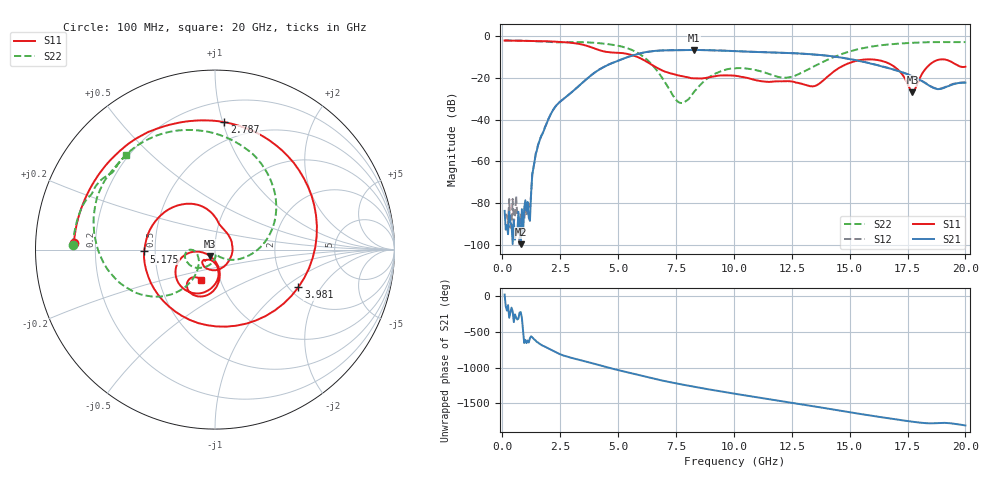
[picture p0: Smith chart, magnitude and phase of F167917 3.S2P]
!  2-Port S-parameters saved by WinCal
! VAR MeasName=S-Parameters (CALIBRATED_DATA) read from VNA (N5242A)
! VAR MeasDate=2016-11-22 8:59:48
! VAR NAME=F167917 3
! VAR FILENAME=F167917 3.S2P
! VAR DATE=2016-11-22 8:59:48
! VAR PHYS_PORTS=1,2
# Hz S DB R 50
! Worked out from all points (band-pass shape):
!   401 points, 100 MHz to 20 GHz, reference 50 ohm
!   highest |S21| = -6.55 dB at 8.259 GHz (marker M1); lowest = -99.6 dB at 796.5 MHz (marker M2)
!   |S21| within 3 dB of the highest: 5.534 GHz to 14.2 GHz (8.669 GHz wide, 87.8 % of centre)
!   lowest |S11| = -26.9 dB at 17.71 GHz (marker M3), VSWR 1.09, Z = 47.1 - j3.3 ohm
!   |S11| at or under -10 dB: 5.847 GHz to end of sweep
!   |S22| runs from -32.0 to -2.0 dB; largest |S21 - S12| = 0.0037
!   S11 on the Smith chart (normalised r, x): 100 MHz: 0.12, +0.02; 2.787 GHz: 0.35, +1.01; 3.981 GHz: 2.24, -1.27; 5.175 GHz: 0.43, -0.01; 20 GHz: 0.81, -0.29
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1e8  -2.09 177.3  -83.65 24.2  -85.98 -168.3  -2.03 178.3
7.965e8  -2.19 158.8  -99.62 138.5  -84.99 84.7  -2.12 166.8
1.14475e9  -2.25 149.1  -87.03 71.5  -80.65 92.5  -2.22 160.8
1.493e9  -2.31 138.7  -54.64 79.0  -54.48 79.8  -2.46 155.5
1.94075e9  -2.42 123.5  -41.01 -2.5  -40.94 -3.9  -2.60 147.9
2.7865e9  -2.95 85.8  -28.76 -125.7  -28.76 -126.2  -2.82 136.0
3.43325e9  -3.95 38.6  -22.54 179.6  -22.57 179.5  -2.86 122.2
3.9805e9  -5.85 -24.3  -17.50 132.0  -17.48 132.1  -3.14 108.0
4.478e9  -7.46 -95.9  -14.23 87.6  -14.17 87.5  -3.66 92.9
5.1745e9  -8.06 -178.5  -10.93 31.1  -10.90 30.6  -4.99 66.1
5.9705e9  -10.61 119.9  -8.14 -31.5  -8.17 -31.9  -8.82 24.4
6.7665e9  -15.64 86.0  -6.87 -92.2  -6.90 -92.3  -17.74 -25.4
7.61225e9  -18.79 56.4  -6.62 -148.4  -6.64 -148.4  -31.57 -72.8
8.259e9  -20.15 7.8  -6.55 172.1  -6.56 172.3  -27.00 -88.3
1.005e10  -18.88 -120.2  -7.12 72.4  -7.12 72.5  -15.35 -157.2
1.159225e10  -21.85 -132.9  -7.74 -6.2  -7.73 -6.2  -18.38 -178.3
1.338325e10  -24.03 -110.9  -8.65 -99.7  -8.65 -99.4  -14.86 -127.8
1.5224e10  -11.99 -106.4  -11.37 161.5  -11.34 161.7  -6.61 -146.9
1.67165e10  -13.16 -160.7  -15.36 87.0  -15.37 87.2  -3.91 -176.3
1.77115e10  -26.88 -129.5  -19.19 40.7  -19.06 40.9  -3.15 166.4
1.87065e10  -11.77 -99.9  -25.09 19.5  -24.94 19.9  -2.81 150.4
2e10  -14.59 -114.0  -22.25 -12.0  -22.08 -12.1  -2.82 133.3
